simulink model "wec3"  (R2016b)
settings: Solver=ode4  StartTime=0  StopTime=500  FixedStep=0.01  MaxStep=0.01  RelTol=1e-3  EnableMultiTasking=on
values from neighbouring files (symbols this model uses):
  arAdaptiveLawData = 1/2*zModelSimple.zModelPto.arFreq.*     zModelSimple.zModelPto.arMagnitude./     cos(zModelSimple.zModelPto.arPhase*pi/180+pi/2)    [IMPACT_Control.m]
  arControllerRampGain = [0,0,1,1]    [IMPACT_Control.m]
  arControllerRampTime = [0 rStartRampTime rStartRampTime+rRampTimeLength 8000]    [IMPACT_Control.m]
  arEkfInitialisation = zeros(1,11)    [IMPACT_Control.m]
  arFrequency = zModelSimple.zModelPto.arFreq    [IMPACT_Control.m]
  arFrequencyRange = zModelSimple.zModelPto.arFreq    [IMPACT_Control.m]
  arImpedance = 1./zModelSimple.zModelPto.arMagnitude./zModelSimple.zModelPto.arFreq    [IMPACT_Control.m]
  arReferenceSpeedGain = [0.949075	0.948701	0.948086	0.947210	0.946078	0.944687	0.943012	0.941068	0.938816	0.936271	0.933396     0.930175	0.926598	0.922654	0.918263	0.913405	0.908086	0.901638	0.895829	0.888757	0.880863	0.872271	0.862778	0.852482     0.840874	0.827739	0.813322	0.797269	0.779501	0.760223	0.737472	0.712445	0.683207	0.651238	0.615591	0.577044	0.538330     0.488567	0.439533	0.392319	0.349558	0.318508	0.304192	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    [wec3AdditionalParams.m]
  iAdaptiveDamping = 0    [wec3_IMPACT_Project.m]    (also in IMPACT_Control.m = handles.iAdaptiveDamping; wec1_IMPACT_Project.m; wec2_IMPACT_Project.m; wec4IMPACT_Project.m)
  iControlType = 1    [wec3_IMPACT_Project.m]    (also in IMPACT_Control.m = handles.iControlType; wec1_IMPACT_Project.m; wec2_IMPACT_Project.m; wec4IMPACT_Project.m = 2)
  iPtoPositionConstraint = 1    [wec3_IMPACT_Project.m]    (also in IMPACT_Control.m = handles.iPtoPositionConstraint; wec1_IMPACT_Project.m = 0; wec2_IMPACT_Project.m; wec4IMPACT_Project.m)
  iSensorNoise = 0    [IMPACT_Control.m]
  m = m+1    (= 2)    [checkParamFile.m]
  rCogFloater = -0.7    [wec3_IMPACT_Model.m]    (also in wec3_IMPACT_Model2.m; paramInitial.m = get( handles.edit_rCogFloater, 'String' ); wec1_IMPACT_Model.m = -18; wec2_IMPACT_Model.m = -8.5)
  rCogSpar = -21.3    [wec3_IMPACT_Model.m]    (also in wec3_IMPACT_Model2.m; paramInitial.m = get( handles.edit_rCogSpar, 'String' ); wec4_IMPACT_Model.m = -36.6)
  rDisplacementLimit = 3.000000    (= 3)    [wec3_IMPACT_Project.m]    (also in IMPACT_Control.m = getValue(handles.edit_displacementLimit); wec1_IMPACT_Project.m = 10; wec2_IMPACT_Project.m = 10; wec4IMPACT_Project.m = 10)
  rGainForAntiWIndUp = tfControllerDiscrete.rGain    [IMPACT_Control.m]
  rMaxForcePto = 1000000000.000000    (= 1000000000)    [wec3_IMPACT_Project.m]    (also in IMPACT_Control.m = getValue(handles.edit_maxForcePto); wec1_IMPACT_Project.m = 1e+15; wec2_IMPACT_Project.m = 1e+15; wec4IMPACT_Project.m = 300000000)
  rMinForcePto = -1000000000.000000    (= -1000000000)    [wec3_IMPACT_Project.m]    (also in IMPACT_Control.m = getValue(handles.edit_minForcePto); wec1_IMPACT_Project.m = -1e+15; wec2_IMPACT_Project.m = -1e+15; wec4IMPACT_Project.m = -300000000)
  rOutputSampleTime = 0.010000    (= 0.01)    [wec3_IMPACT_Project.m]    (also in IMPACT_Control.m = getValue(handles.edit_outputSampleTime); wec1_IMPACT_Project.m; wec2_IMPACT_Project.m; wec4IMPACT_Project.m)
  rPassiveDampingGain = -519390.000000    (= -519390)    [wec3_IMPACT_Project.m]    (also in IMPACT_Control.m = getValue(handles.edit_gainPLD); wec1_IMPACT_Project.m = -214018.1537; wec2_IMPACT_Project.m = -1948070; wec4IMPACT_Project.m = -604830)
  s = tf('s')    [wec3_IMPACT_Model.m]    (also in wec3_IMPACT_Model2.m; IMPACT_Control.m; wec1_IMPACT_Model.m; wec2_IMPACT_Model.m)
  simu = simulationClass()    [wecSimInputFile.m]
  Z = magPhaseToComplex(zModelTf)    [IMPACT_Control.m]
undefined symbols (not defined in the file or in its folder): arControllerDiscreteDen, arControllerDiscreteNum, arExcForceFloaterDen, arExcForceFloaterNum, arExcForceSparDen, arExcForceSparNum, arFexcFloaterDen, arFexcFloaterNum, arFexcSparDen, arFexcSparNum, arRefeneceSpeedFreq, body, constraint, magnitude, mooring, N, pto, rAccelerationGainFloater, rAccelerationGainSpar, rBuoyancyGainFloater, rBuoyancyGainSpar, rDampingGainFloater, rDampingGainSpar, X, Y
libraries: nesl_utility x9, simulink x6, WECSim_Lib x5, sm_lib x5

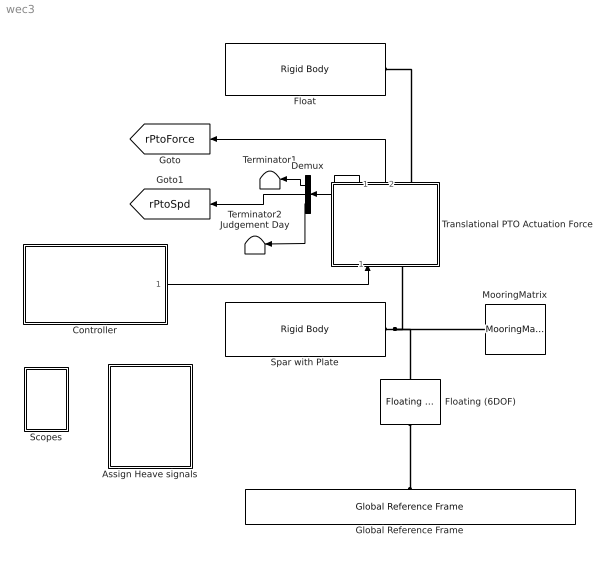
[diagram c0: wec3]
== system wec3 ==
  Assign Heave signals : Subsystem
  Controller : Subsystem
  Demux : Demux  Outputs=3
  Float : WECSim_Lib/Body Elements/Rigid Body  body=body(1)
  Floating (6DOF) : WECSim_Lib/Constraints/Floating (6DOF)  constraint=constraint(1)
  Global Reference Frame : WECSim_Lib/Frames/Global Reference Frame  waves=waves  simu=simu
  MooringMatrix : WECSim_Lib/Moorings/MooringMatrix  mooring=mooring(1)
  Scopes : Subsystem
  Spar with Plate : WECSim_Lib/Body Elements/Rigid Body  body=body(2)
  Terminator1 : Terminator
  Terminator2 Judgement Day : Terminator
  Translational PTO Actuation Force : Subsystem  AncestorBlock=WECSim_Lib/PTOs/Translational PTO Actuation Force
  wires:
  Translational PTO Actuation Force/2(ptoForce) -> [rPtoForce]
  Controller/1(forceDemandOut) -> Translational PTO Actuation Force/1(Force)
  Translational PTO Actuation Force/1(Response) -> Demux/1
  Demux/2 -> [rPtoSpd]
  Demux/1 -> Terminator1/1
  Demux/3 -> Terminator2 Judgement Day/1
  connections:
  Spar with Plate/RConn1 -- Translational PTO Actuation Force/LConn1 -- Floating (6DOF)/RConn1 -- MooringMatrix/LConn1
  Translational PTO Actuation Force/RConn1 -- Float/RConn1
  Floating (6DOF)/LConn1 -- Global Reference Frame/RConn1

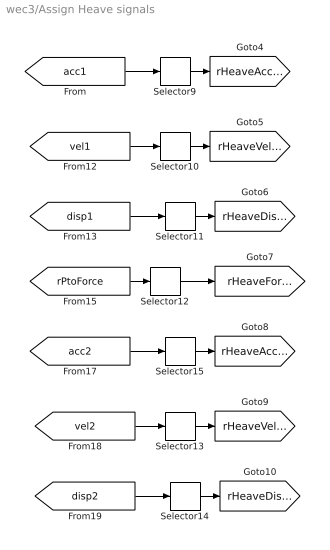
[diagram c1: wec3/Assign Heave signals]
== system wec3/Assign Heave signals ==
  Selector{9..15} (7 alike) : Selector  InputPortWidth=6  IndexOptions=Index vector (dialog)  Indices=3  OutputSizes=1
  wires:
  Selector11/1 -> [rHeaveDispFl]
  [disp1] -> Selector11/1
  Selector12/1 -> [rHeaveForcePto]
  [vel1] -> Selector10/1
  [acc1] -> Selector9/1
  Selector10/1 -> [rHeaveVelFl]
  Selector9/1 -> [rHeaveAccFl]
  [rPtoForce] -> Selector12/1
  Selector14/1 -> [rHeaveDispSp]
  Selector13/1 -> [rHeaveVelSp]
  [vel2] -> Selector13/1
  [disp2] -> Selector14/1
  [acc2] -> Selector15/1
  Selector15/1 -> [rHeaveAccSp]

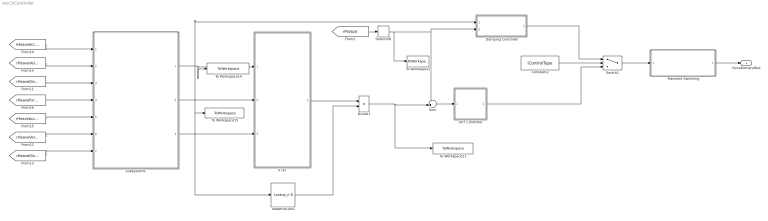
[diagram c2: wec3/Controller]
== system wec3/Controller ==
  Constant2 : Constant  Value=iControlType
  Damping Controller : Subsystem
  Divide1 : Product  Inputs=**
  OVT Controller : Subsystem
  Selector6 : Selector  InputPortWidth=6  IndexOptions=Index vector (dialog)  Indices=3  OutputSizes=1
  Subsystem1 : Subsystem
  Sum : Sum  Inputs=-+|
  Switch1 : Switch  Threshold=2
  To Workspace14 : ToWorkspace  VariableName=arCombinedExcForce  SampleTime=simu.dtOut
  To Workspace15 : ToWorkspace  VariableName=arFreqCombExcF  SampleTime=simu.dtOut
  To Workspace2 : ToWorkspace  VariableName=arPtoVelocity  SampleTime=0.05
  To Workspace21 : ToWorkspace  VariableName=arReferenceVelocity  SampleTime=simu.dtOut
  Transient Switching : Subsystem
  "V ref " : Subsystem
  adaptiveLaw1 : Lookup_n-D  NumberOfTableDimensions=1  BreakpointsForDimension1=arRefeneceSpeedFreq  Table=arReferenceSpeedGain  InternalRulePriority=Speed  RndMeth=Simplest
  forceDemandOut : Outport
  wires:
  [rHeaveDispSp] -> Subsystem1/7(sparPos)
  [rHeaveVelFl] -> Subsystem1/2(floaterVel)
  [rHeaveAccFl] -> Subsystem1/1(floaterAcc)
  [rHeaveAccSp] -> Subsystem1/5(sparAcc)
  [rHeaveVelSp] -> Subsystem1/6(sparVel)
  [rHeaveForcePto] -> Subsystem1/4(ptoForce)
  [rHeaveDispFl] -> Subsystem1/3(floaterPos)
  Damping Controller/1(forceDemand) -> Switch1/1
  Switch1/1 -> Transient Switching/1(forceDemandIn)
  Constant2/1 -> Switch1/2
  OVT Controller/1(forceDemand) -> Switch1/3
  Sum/1 -> OVT Controller/1(error)
  Selector6/1 -> To Workspace2/1, Sum/1, Damping Controller/2(velocity)
  [rPtoSpd] -> Selector6/1
  Subsystem1/2(Frequency) -> adaptiveLaw1/1, To Workspace15/1, "V ref "/2(ekfFrequency), Damping Controller/1(ekfFrequency)
  Subsystem1/3(Exc. Force Amplitude) -> "V ref "/3(ekfAmplitude)
  Subsystem1/1(Combined Excitation Force) -> To Workspace14/1, "V ref "/1(phiOut)
  Transient Switching/1(forceDemandOut) -> forceDemandOut/1
  "V ref "/1(referenceVelocity) -> Divide1/1
  adaptiveLaw1/1 -> Divide1/2
  Divide1/1 -> To Workspace21/1, Sum/2

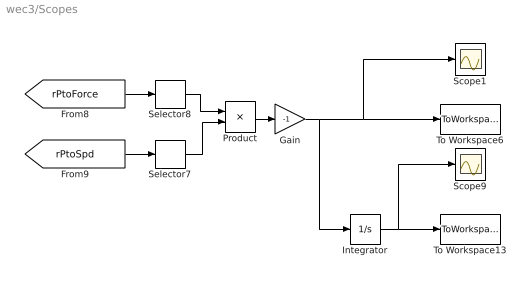
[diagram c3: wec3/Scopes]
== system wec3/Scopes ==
  Gain : Gain  Gain=-1
  Integrator : Integrator
  Product : Product
  Scope1 : Scope
  Scope9 : Scope
  Selector7 : Selector  InputPortWidth=6  IndexOptions=Index vector (dialog)  Indices=3  OutputSizes=1
  Selector8 : Selector  InputPortWidth=6  IndexOptions=Index vector (dialog)  Indices=3  OutputSizes=1
  To Workspace13 : ToWorkspace  VariableName=arWecEnergy  SampleTime=simu.dtOut
  To Workspace6 : ToWorkspace  VariableName=arWecPower  SampleTime=simu.dtOut
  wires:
  Gain/1 -> To Workspace6/1, Scope1/1, Integrator/1
  [rPtoForce] -> Selector8/1
  [rPtoSpd] -> Selector7/1
  Product/1 -> Gain/1
  Selector7/1 -> Product/2
  Selector8/1 -> Product/1
  Integrator/1 -> Scope9/1, To Workspace13/1

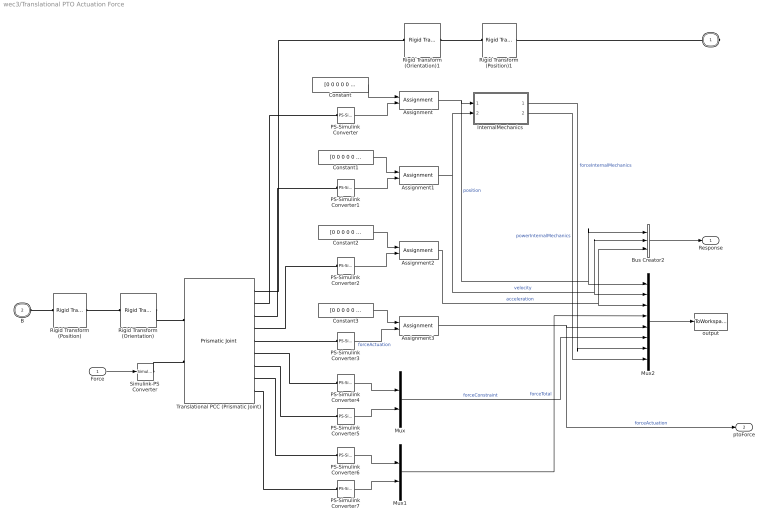
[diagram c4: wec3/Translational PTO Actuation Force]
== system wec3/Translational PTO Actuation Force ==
  Force : Inport
  Assignment{,1..3} (4 alike) : Assignment  IndexOptions=Index vector (dialog)  Indices=3  OutputSizes=1
  Bus Creator2 : BusCreator  Inputs=3
  Constant{,1..3} (4 alike) : Constant  Value=[0 0 0 0 0 0]
  InternalMechanics : Subsystem
  Mux : Mux  Inputs=2
  Mux1 : Mux  Inputs=2
  Mux2 : Mux  Inputs=8
  PS-Simulink Converter{,1..7} (8 alike) : nesl_utility/PS-Simulink Converter  PhysicalDomain=network_engine_domain  SubClassName=ps_output  LeftPortType=input  RightPortType=output  PseudoPeriodic=off  Frequencies=[]  Unit=1  AffineConversion=off
  Rigid Transform (Position) : sm_lib/Frames and Transforms/Rigid Transform  TranslationMethod=Cartesian  TranslationStandardOffset=0  TranslationLengthUnit=m  TranslationStandardAxis=+Z  TranslationCartesianOffset=pto.initDisp.initLinDisp + pto.loc  TranslationROffset=0  TranslationROffsetUnits=m  TranslationZOffset=0  TranslationZOffsetUnits=m  TranslationThetaOffset=0  TranslationThetaOffsetUnits=deg  RotationMethod=None  RotationAngleUnits=rad  RotationStandardAxis=+Y  RotationAngle=0  RotationArbitraryAxis=[0 1 0]  FollAlignAxisA=+X  BaseAlignAxisA=+Y  FollAlignAxisB=+Y  BaseAlignAxisB=+Z  RotationSequenceAxes=FollowerAxes  RotationSequence=XYX  RotationSequenceAngles=[0 0 0]  RotationSequenceAnglesUnits=deg  RotationMatrix=[1 0 0; 0 1 0; 0 0 1]
  Rigid Transform (Position)1 : sm_lib/Frames and Transforms/Rigid Transform  TranslationMethod=Cartesian  TranslationStandardOffset=0  TranslationLengthUnit=m  TranslationStandardAxis=+Z  TranslationCartesianOffset=pto.initDisp.initLinDisp + pto.loc  TranslationROffset=0  TranslationROffsetUnits=m  TranslationZOffset=0  TranslationZOffsetUnits=m  TranslationThetaOffset=0  TranslationThetaOffsetUnits=deg  RotationMethod=None  RotationAngleUnits=rad  RotationStandardAxis=+Y  RotationAngle=0  RotationArbitraryAxis=[0 1 0]  FollAlignAxisA=+X  BaseAlignAxisA=+Y  FollAlignAxisB=+Y  BaseAlignAxisB=+Z  RotationSequenceAxes=FollowerAxes  RotationSequence=XYX  RotationSequenceAngles=[0 0 0]  RotationSequenceAnglesUnits=deg  RotationMatrix=[1 0 0; 0 1 0; 0 0 1]
  Rigid Transform (Orientation) : sm_lib/Frames and Transforms/Rigid Transform  TranslationMethod=None  TranslationStandardOffset=0  TranslationLengthUnit=m  TranslationStandardAxis=+Z  TranslationCartesianOffset=0  TranslationROffset=0  TranslationROffsetUnits=m  TranslationZOffset=0  TranslationZOffsetUnits=m  TranslationThetaOffset=0  TranslationThetaOffsetUnits=deg  RotationMethod=RotationMatrix  RotationAngleUnits=rad  RotationStandardAxis=+Y  RotationAngle=0  RotationArbitraryAxis=[0 1 0]  FollAlignAxisA=+X  BaseAlignAxisA=+Y  FollAlignAxisB=+Y  BaseAlignAxisB=+Z  RotationSequenceAxes=FollowerAxes  RotationSequence=XYX  RotationSequenceAngles=[0 0 0]  RotationSequenceAnglesUnits=deg  RotationMatrix=pto.orientation.rotationMatrix
  Rigid Transform (Orientation)1 : sm_lib/Frames and Transforms/Rigid Transform  TranslationMethod=None  TranslationStandardOffset=0  TranslationLengthUnit=m  TranslationStandardAxis=+Z  TranslationCartesianOffset=0  TranslationROffset=0  TranslationROffsetUnits=m  TranslationZOffset=0  TranslationZOffsetUnits=m  TranslationThetaOffset=0  TranslationThetaOffsetUnits=deg  RotationMethod=RotationMatrix  RotationAngleUnits=rad  RotationStandardAxis=+Y  RotationAngle=0  RotationArbitraryAxis=[0 1 0]  FollAlignAxisA=+X  BaseAlignAxisA=+Y  FollAlignAxisB=+Y  BaseAlignAxisB=+Z  RotationSequenceAxes=FollowerAxes  RotationSequence=XYX  RotationSequenceAngles=[0 0 0]  RotationSequenceAnglesUnits=deg  RotationMatrix=pto.orientation.rotationMatrix
  Simulink-PS Converter : nesl_utility/Simulink-PS Converter  PhysicalDomain=network_engine_domain  SubClassName=ps_input  LeftPortType=input  RightPortType=output  PseudoPeriodic=off  Frequencies=[]  NoiseDistribution=none  NoiseParameters=[]  Unit=1  AffineConversion=off  InputFiltering=off  SimscapeFilterOrder=1  InputFilterTimeConstant=0.001  UdotUserProvided=1
  Translational PCC (Prismatic Joint) : sm_lib/Joints/Prismatic Joint  SenseConstraintForce=on  SenseConstraintForceX=off  SenseConstraintForceY=off  SenseConstraintForceZ=off  SenseConstraintTorque=on  SenseConstraintTorqueX=off  SenseConstraintTorqueY=off  SenseConstraintTorqueZ=off  SenseTotalForce=on  SenseTotalForceX=off  SenseTotalForceY=off  SenseTotalForceZ=off  SenseTotalTorque=on  SenseTotalTorqueX=off  SenseTotalTorqueY=off  SenseTotalTorqueZ=off  CompositeWrenchDir=BaseOnFollower  CompositeWrenchFrame=BaseFrame  EquilibriumPosition=0  EquilibriumPositionUnits=m  SpringStiffness=pto.k  SpringStiffnessUnits=N/m  DampingCoefficient=pto.c  DampingCoefficientUnits=N/(m/s)  TorqueActuationMode=InputTorque  MotionActuationMode=ComputedMotion  SensePosition=on  SenseVelocity=on  SenseAcceleration=on  SenseTorqueForce=on  PositionTargetSpecify=off  PositionTargetPriority=High  PositionTargetValue=0  PositionTargetValueUnits=m  VelocityTargetSpecify=off  VelocityTargetPriority=High  VelocityTargetValue=0  VelocityTargetValueUnits=m/s
  output : ToWorkspace  VariableName=pto1_out  SaveFormat=Structure With Time  SampleTime=-1
  F : PMIOPort  Port=1  Side=Right
  B : PMIOPort  Port=2  Side=Left
  Response : Outport
  ptoForce : Outport  Port=2
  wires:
  Bus Creator2/1 -> Response/1
  Assignment/1 -> Mux2/1, Bus Creator2/1, InternalMechanics/1(Position)  "position"
  Assignment1/1 -> Mux2/2, Bus Creator2/2, InternalMechanics/2(Velocity)  "velocity"
  Assignment2/1 -> Mux2/3, Bus Creator2/3  "acceleration"
  Force/1 -> Simulink-PS Converter/1
  Mux2/1 -> output/1
  Mux/1 -> Mux2/6  "forceConstraint"
  Mux1/1 -> Mux2/4  "forceTotal"
  PS-Simulink Converter4/1 -> Mux/1
  PS-Simulink Converter5/1 -> Mux/2
  PS-Simulink Converter6/1 -> Mux1/1
  PS-Simulink Converter7/1 -> Mux1/2
  Assignment3/1 -> ptoForce/1, Mux2/5  "forceActuation"
  Constant/1 -> Assignment/1
  PS-Simulink Converter/1 -> Assignment/2
  Constant1/1 -> Assignment1/1
  PS-Simulink Converter1/1 -> Assignment1/2
  Constant2/1 -> Assignment2/1
  PS-Simulink Converter2/1 -> Assignment2/2
  InternalMechanics/1(Force) -> Mux2/7  "forceInternalMechanics"
  InternalMechanics/2(Power) -> Mux2/8  "powerInternalMechanics"
  Constant3/1 -> Assignment3/1
  PS-Simulink Converter3/1 -> Assignment3/2  "forceActuation"
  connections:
  Rigid Transform (Position)/RConn1 -- Rigid Transform (Orientation)/LConn1
  Rigid Transform (Position)1/RConn1 -- Rigid Transform (Orientation)1/LConn1
  Simulink-PS Converter/RConn1 -- Translational PCC (Prismatic Joint)/LConn2
  Rigid Transform (Orientation)/RConn1 -- Translational PCC (Prismatic Joint)/LConn1
  Rigid Transform (Position)/LConn1 -- B/RConn1
  Translational PCC (Prismatic Joint)/RConn5 -- PS-Simulink Converter3/LConn1
  Translational PCC (Prismatic Joint)/RConn9 -- PS-Simulink Converter7/LConn1
  Rigid Transform (Orientation)1/RConn1 -- Translational PCC (Prismatic Joint)/RConn1
  Translational PCC (Prismatic Joint)/RConn4 -- PS-Simulink Converter2/LConn1
  Translational PCC (Prismatic Joint)/RConn7 -- PS-Simulink Converter5/LConn1
  Translational PCC (Prismatic Joint)/RConn3 -- PS-Simulink Converter1/LConn1
  Rigid Transform (Position)1/LConn1 -- F/RConn1
  Translational PCC (Prismatic Joint)/RConn8 -- PS-Simulink Converter6/LConn1
  Translational PCC (Prismatic Joint)/RConn2 -- PS-Simulink Converter/LConn1
  Translational PCC (Prismatic Joint)/RConn6 -- PS-Simulink Converter4/LConn1

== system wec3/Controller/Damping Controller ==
  ekfFrequency : Inport
  velocity : Inport  Port=2
  Constant2 : Constant  Value=iAdaptiveDamping
  Divide2 : Product  Inputs=**
  Gain6 : Gain  Gain=rPassiveDampingGain
  Gain7 : Gain  Gain=-1
  Switch1 : Switch  Criteria=u2 > Threshold
  adaptiveLaw1 : Lookup_n-D  NumberOfTableDimensions=1  BreakpointsForDimension1=arFrequency  Table=arImpedance  InternalRulePriority=Speed  RndMeth=Simplest
  forceDemand : Outport
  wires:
  Divide2/1 -> Switch1/1
  ekfFrequency/1 -> adaptiveLaw1/1
  adaptiveLaw1/1 -> Gain7/1
  Constant2/1 -> Switch1/2
  Switch1/1 -> forceDemand/1
  Gain7/1 -> Divide2/1
  velocity/1 -> Divide2/2, Gain6/1
  Gain6/1 -> Switch1/3

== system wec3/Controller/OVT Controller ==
  error : Inport
  Anti wind-up controller : Subsystem
  forceDemand : Outport
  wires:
  error/1 -> Anti wind-up controller/1(error)
  Anti wind-up controller/1(Out1) -> forceDemand/1

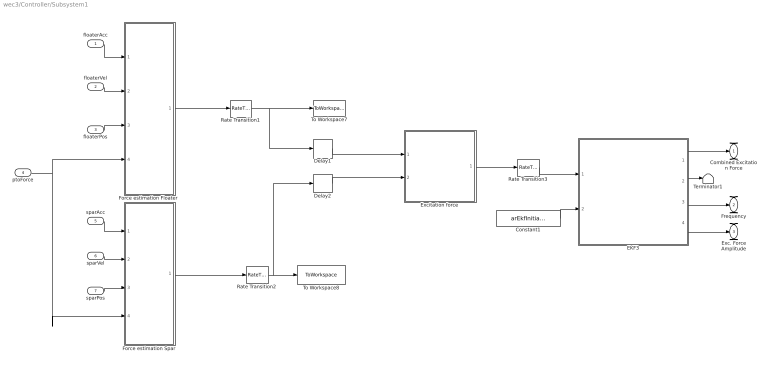
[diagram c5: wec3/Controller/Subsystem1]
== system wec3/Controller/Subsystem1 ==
  floaterAcc : Inport
  floaterVel : Inport  Port=2
  floaterPos : Inport  Port=3
  ptoForce : Inport  Port=4
  sparAcc : Inport  Port=5
  sparVel : Inport  Port=6
  sparPos : Inport  Port=7
  Constant1 : Constant  Value=arEkfInitialisation
  Delay1 : Delay  DelayLength=1  SampleTime=simu.dt
  Delay2 : Delay  DelayLength=1  SampleTime=simu.dt
  EKF3 : MATLAB Function  TreatAsAtomicUnit=on
  Excitation force : Subsystem
  "Force estimation Floater " : Subsystem
  Force estimation Spar : Subsystem
  Rate Transition1 : RateTransition  OutPortSampleTimeMultiple=0.01  OutPortSampleTime=rKalmanFilterSampleTime
  Rate Transition2 : RateTransition  OutPortSampleTimeMultiple=0.01  OutPortSampleTime=rKalmanFilterSampleTime
  Rate Transition3 : RateTransition  OutPortSampleTimeMultiple=0.01  OutPortSampleTime=rKalmanFilterSampleTime
  Terminator1 : Terminator
  To Workspace7 : ToWorkspace  VariableName=arExcForceFl  SampleTime=simu.dtOut
  To Workspace8 : ToWorkspace  VariableName=arExcForceSp  SampleTime=simu.dtOut
  Combined Excitation Force : Outport
  Frequency : Outport  Port=2
  Exc. Force Amplitude : Outport  Port=3
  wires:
  Excitation force/1(Combined Fexc) -> Rate Transition3/1
  Rate Transition2/1 -> Delay2/1, To Workspace8/1
  ptoForce/1 -> Force estimation Spar/4(PTO Force), "Force estimation Floater "/4(PTO force)
  floaterVel/1 -> "Force estimation Floater "/2(Velocity)
  sparVel/1 -> Force estimation Spar/2(Velocity)
  Rate Transition1/1 -> To Workspace7/1, Delay1/1
  sparAcc/1 -> Force estimation Spar/1(Acceleration)
  sparPos/1 -> Force estimation Spar/3(Position)
  floaterAcc/1 -> "Force estimation Floater "/1(Acceleration)
  floaterPos/1 -> "Force estimation Floater "/3(Position)
  "Force estimation Floater "/1(excForce) -> Rate Transition1/1
  Force estimation Spar/1(excForce) -> Rate Transition2/1
  Rate Transition3/1 -> EKF3/1(rEstimatedExcitationForce)
  EKF3/3(rFrequencyOutput) -> Frequency/1
  EKF3/4(rAmplitudeOutput) -> Exc. Force Amplitude/1
  EKF3/1(rPhi0Output) -> Combined Excitation Force/1
  Constant1/1 -> EKF3/2(arEkfInitialisation)
  EKF3/2(rPhi0StarOutput) -> Terminator1/1
  Delay1/1 -> Excitation force/1(Fexc floater)
  Delay2/1 -> Excitation force/2(Fexc spar)

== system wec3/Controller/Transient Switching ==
  forceDemandIn : Inport
  Constant : Constant
  IC : InitialCondition  Value=0
  Product : Product
  To Workspace3 : ToWorkspace  VariableName=arForceDemand  SampleTime=rOutputSampleTime
  To Workspace7 : ToWorkspace  VariableName=arForceDemandIn  SampleTime=rOutputSampleTime
  forceDemandOut : Outport
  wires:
  forceDemandIn/1 -> Product/2, To Workspace7/1
  Product/1 -> IC/1
  IC/1 -> To Workspace3/1, forceDemandOut/1
  Constant/1 -> Product/1

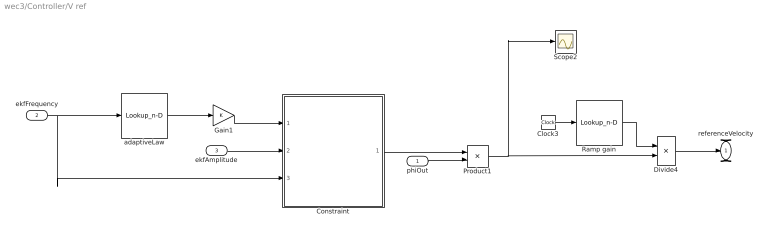
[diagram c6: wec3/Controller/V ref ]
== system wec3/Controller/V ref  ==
  phiOut : Inport
  ekfFrequency : Inport  Port=2
  ekfAmplitude : Inport  Port=3
  Clock3 : Clock
  Constraint : Subsystem
  Divide4 : Product  Inputs=**
  Gain1 : Gain
  Product1 : Product
  Ramp gain : Lookup_n-D  NumberOfTableDimensions=1  BreakpointsForDimension1=arControllerRampTime  Table=arControllerRampGain  InternalRulePriority=Speed  RndMeth=Simplest
  Scope2 : Scope
  adaptiveLaw : Lookup_n-D  NumberOfTableDimensions=1  BreakpointsForDimension1=arFrequencyRange  Table=arAdaptiveLawData  InternalRulePriority=Speed  RndMeth=Simplest
  referenceVelocity : Outport
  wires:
  Constraint/1(referenceVelocity) -> Product1/1
  Ramp gain/1 -> Divide4/1
  Clock3/1 -> Ramp gain/1
  Gain1/1 -> Constraint/1(1/2B)
  adaptiveLaw/1 -> Gain1/1
  Divide4/1 -> referenceVelocity/1
  ekfFrequency/1 -> Constraint/3(ekfFrequency), adaptiveLaw/1
  ekfAmplitude/1 -> Constraint/2(Amp)
  Product1/1 -> Scope2/1, Divide4/2
  phiOut/1 -> Product1/2

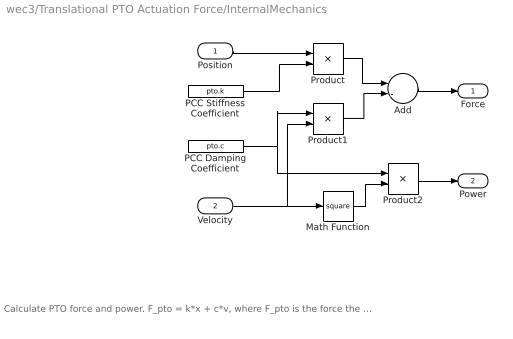
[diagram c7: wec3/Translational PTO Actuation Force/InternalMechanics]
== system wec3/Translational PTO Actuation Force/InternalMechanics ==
  note: Calculate PTO force and power. F_pto = k*x + c*v, where F_pto is the force the PTO applies to the body (at the PTO location), x and v are the joint position and velocity. The power extracted is P = c * v^2
  Position : Inport
  Velocity : Inport  Port=2
  Add : Sum  Inputs=--
  Math Function : Math  Operator=square
  PCC Damping Coefficient : Constant  Value=pto.c
  PCC Stiffness Coefficient : Constant  Value=pto.k
  Product : Product  Inputs=**
  Product1 : Product  Inputs=**
  Product2 : Product  Inputs=**
  Force : Outport
  Power : Outport  Port=2
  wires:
  PCC Damping Coefficient/1 -> Product2/1, Product1/1
  Product2/1 -> Power/1
  Velocity/1 -> Math Function/1, Product1/2
  PCC Stiffness Coefficient/1 -> Product/2
  Position/1 -> Product/1
  Add/1 -> Force/1
  Math Function/1 -> Product2/2
  Product/1 -> Add/1
  Product1/1 -> Add/2

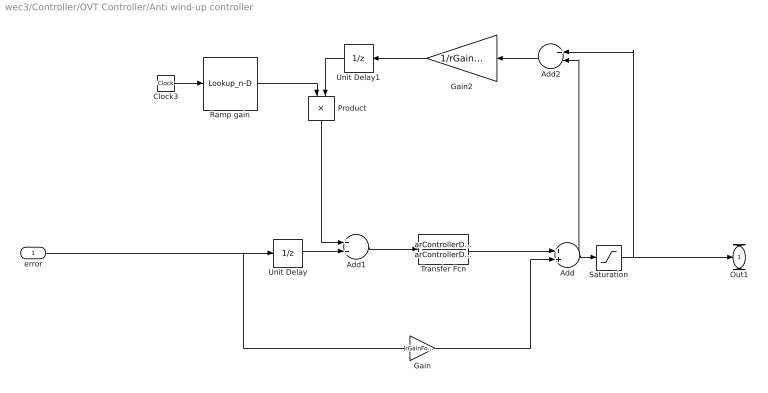
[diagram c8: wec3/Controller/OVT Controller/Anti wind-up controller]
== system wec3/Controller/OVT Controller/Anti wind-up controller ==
  error : Inport
  Add : Sum
  Add1 : Sum
  Add2 : Sum  Inputs=+-
  Clock3 : Clock
  Gain : Gain  Gain=rGainForAntiWIndUp
  Gain2 : Gain  Gain=1/rGainForAntiWIndUp
  Product : Product
  Ramp gain : Lookup_n-D  NumberOfTableDimensions=1  BreakpointsForDimension1=arControllerRampTime  Table=arControllerRampGain  InternalRulePriority=Speed  RndMeth=Simplest
  Saturation : Saturate  UpperLimit=rMaxForcePto  LowerLimit=rMinForcePto
  Transfer Fcn : TransferFcn  Numerator=arControllerDiscreteNum  Denominator=arControllerDiscreteDen
  Unit Delay : UnitDelay  SampleTime=0.01
  Unit Delay1 : UnitDelay  SampleTime=0.01
  Out1 : Outport
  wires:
  Add/1 -> Saturation/1, Add2/2
  Gain/1 -> Add/2
  Unit Delay/1 -> Add1/2
  Gain2/1 -> Unit Delay1/1
  error/1 -> Gain/1, Unit Delay/1
  Add2/1 -> Gain2/1
  Add1/1 -> Transfer Fcn/1
  Clock3/1 -> Ramp gain/1
  Ramp gain/1 -> Product/1
  Product/1 -> Add1/1
  Unit Delay1/1 -> Product/2
  Saturation/1 -> Out1/1, Add2/1
  Transfer Fcn/1 -> Add/1

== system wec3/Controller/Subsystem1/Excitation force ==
  Fexc floater : Inport
  Fexc spar : Inport  Port=2
  Add : Sum
  Scope : Scope
  Scope1 : Scope
  Scope2 : Scope
  Transfer Fcn : TransferFcn  Numerator=arFexcFloaterNum  Denominator=arFexcFloaterDen
  Transfer Fcn1 : TransferFcn  Numerator=arFexcSparNum  Denominator=arFexcSparDen
  Combined Fexc : Outport
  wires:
  Fexc floater/1 -> Transfer Fcn/1
  Fexc spar/1 -> Transfer Fcn1/1
  Transfer Fcn/1 -> Add/1, Scope1/1
  Transfer Fcn1/1 -> Add/2, Scope2/1
  Add/1 -> Combined Fexc/1, Scope/1

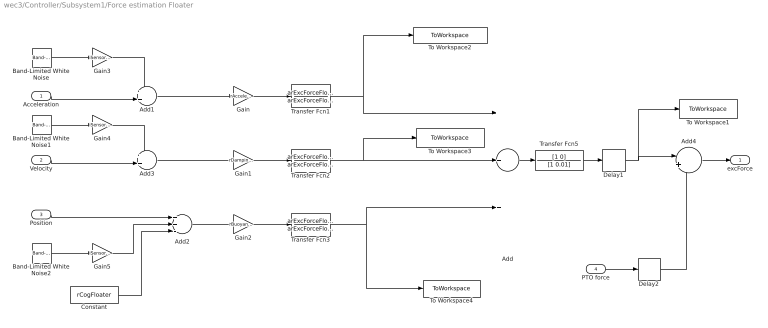
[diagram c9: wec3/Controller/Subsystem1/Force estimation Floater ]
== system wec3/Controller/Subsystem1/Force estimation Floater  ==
  Acceleration : Inport
  Velocity : Inport  Port=2
  Position : Inport  Port=3
  PTO force : Inport  Port=4
  Add : Sum  Inputs=+++
  Add1 : Sum  Inputs=++|
  Add2 : Sum  Inputs=++-
  Add3 : Sum  Inputs=++|
  Add4 : Sum  Inputs=|+-
  Band-Limited White Noise : simulink/Sources/Band-Limited White Noise  Cov=[0.1]  Ts=simu.dt  seed=[23341]
  Band-Limited White Noise1 : simulink/Sources/Band-Limited White Noise  Cov=[0.1]  Ts=simu.dt  seed=[23341]
  Band-Limited White Noise2 : simulink/Sources/Band-Limited White Noise  Cov=[0.1]  Ts=simu.dt  seed=[23341]
  Constant : Constant  Value=rCogFloater
  Delay1 : Delay  DelayLength=1  SampleTime=simu.dt
  Delay2 : Delay  DelayLength=1  SampleTime=simu.dt
  Gain : Gain  Gain=rAccelerationGainFloater
  Gain1 : Gain  Gain=rDampingGainFloater
  Gain2 : Gain  Gain=rBuoyancyGainFloater
  Gain3 : Gain  Gain=iSensorNoise
  Gain4 : Gain  Gain=iSensorNoise
  Gain5 : Gain  Gain=iSensorNoise
  To Workspace1 : ToWorkspace  VariableName=arInertialForceFl  SampleTime=rOutputSampleTime
  To Workspace2 : ToWorkspace  VariableName=arAccComponentFl  SampleTime=rOutputSampleTime
  To Workspace3 : ToWorkspace  VariableName=arVelComponentFl  SampleTime=rOutputSampleTime
  To Workspace4 : ToWorkspace  VariableName=arPosComponentFl  SampleTime=rOutputSampleTime
  Transfer Fcn1 : TransferFcn  Numerator=arExcForceFloaterNum  Denominator=arExcForceFloaterDen
  Transfer Fcn2 : TransferFcn  Numerator=arExcForceFloaterNum  Denominator=arExcForceFloaterDen
  Transfer Fcn3 : TransferFcn  Numerator=arExcForceFloaterNum  Denominator=arExcForceFloaterDen
  Transfer Fcn5 : TransferFcn  Numerator=[1 0]  Denominator=[1 0.01]
  excForce : Outport
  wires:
  Acceleration/1 -> Add1/2
  Band-Limited White Noise/1 -> Gain3/1
  Gain5/1 -> Add2/2
  Add2/1 -> Gain2/1
  Gain2/1 -> Transfer Fcn3/1
  Gain1/1 -> Transfer Fcn2/1
  Gain/1 -> Transfer Fcn1/1
  Constant/1 -> Add2/3
  Gain4/1 -> Add3/1
  Add3/1 -> Gain1/1
  Gain3/1 -> Add1/1
  Velocity/1 -> Add3/2
  Add1/1 -> Gain/1
  Position/1 -> Add2/1
  Band-Limited White Noise1/1 -> Gain4/1
  Band-Limited White Noise2/1 -> Gain5/1
  Add4/1 -> excForce/1
  PTO force/1 -> Delay2/1
  Delay2/1 -> Add4/2
  Delay1/1 -> To Workspace1/1, Add4/1
  Transfer Fcn1/1 -> To Workspace2/1, Add/1
  Transfer Fcn2/1 -> To Workspace3/1, Add/2
  Transfer Fcn3/1 -> To Workspace4/1, Add/3
  Transfer Fcn5/1 -> Delay1/1
  Add/1 -> Transfer Fcn5/1

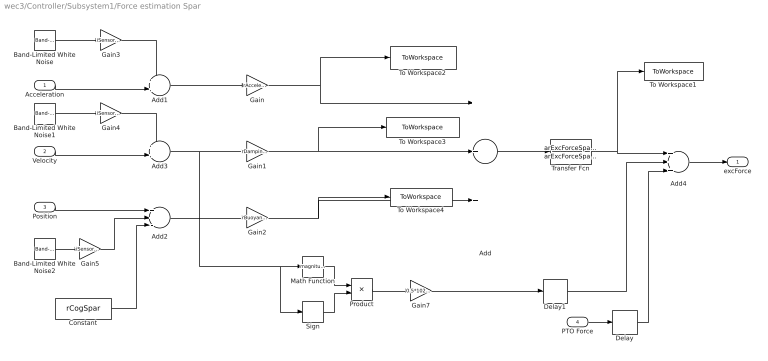
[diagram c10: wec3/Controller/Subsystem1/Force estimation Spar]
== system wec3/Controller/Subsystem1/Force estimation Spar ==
  Acceleration : Inport
  Velocity : Inport  Port=2
  Position : Inport  Port=3
  PTO Force : Inport  Port=4
  Add : Sum  Inputs=+++
  Add1 : Sum  Inputs=++|
  Add2 : Sum  Inputs=++-
  Add3 : Sum  Inputs=++|
  Add4 : Sum  Inputs=+++
  Band-Limited White Noise : simulink/Sources/Band-Limited White Noise  Cov=[0.1]  Ts=simu.dt  seed=[23341]
  Band-Limited White Noise1 : simulink/Sources/Band-Limited White Noise  Cov=[0.1]  Ts=simu.dt  seed=[23341]
  Band-Limited White Noise2 : simulink/Sources/Band-Limited White Noise  Cov=[0.1]  Ts=simu.dt  seed=[23341]
  Constant : Constant  Value=rCogSpar
  Delay : Delay  DelayLength=1  SampleTime=simu.dt
  Delay1 : Delay  DelayLength=1  SampleTime=simu.dt
  Gain : Gain  Gain=rAccelerationGainSpar
  Gain1 : Gain  Gain=rDampingGainSpar
  Gain2 : Gain  Gain=rBuoyancyGainSpar
  Gain3 : Gain  Gain=iSensorNoise
  Gain4 : Gain  Gain=iSensorNoise
  Gain5 : Gain  Gain=iSensorNoise
  Gain7 : Gain  Gain=0.5*1025*pi*15^2*4
  Math Function : Math  Operator=magnitude^2
  Product : Product
  Sign : Signum
  To Workspace1 : ToWorkspace  VariableName=arInertialForceSp  SampleTime=rOutputSampleTime
  To Workspace2 : ToWorkspace  VariableName=arAccComponentSp  SampleTime=rOutputSampleTime
  To Workspace3 : ToWorkspace  VariableName=arVelComponentSp  SampleTime=rOutputSampleTime
  To Workspace4 : ToWorkspace  VariableName=arPosComponentSp  SampleTime=rOutputSampleTime
  Transfer Fcn : TransferFcn  Numerator=arExcForceSparNum  Denominator=arExcForceSparDen
  excForce : Outport
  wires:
  Transfer Fcn/1 -> To Workspace1/1, Add4/1
  Add4/1 -> excForce/1
  Add/1 -> Transfer Fcn/1
  Delay/1 -> Add4/3
  Band-Limited White Noise2/1 -> Gain5/1
  Band-Limited White Noise1/1 -> Gain4/1
  Position/1 -> Add2/1
  Add1/1 -> Gain/1
  Velocity/1 -> Add3/2
  Gain3/1 -> Add1/1
  Add3/1 -> Sign/1, Math Function/1, Gain1/1
  Gain4/1 -> Add3/1
  Constant/1 -> Add2/3
  Gain/1 -> To Workspace2/1, Add/1
  Gain1/1 -> To Workspace3/1, Add/2
  Gain2/1 -> To Workspace4/1, Add/3
  PTO Force/1 -> Delay/1
  Add2/1 -> Gain2/1
  Gain5/1 -> Add2/2
  Band-Limited White Noise/1 -> Gain3/1
  Acceleration/1 -> Add1/2
  Math Function/1 -> Product/1
  Sign/1 -> Product/2
  Product/1 -> Gain7/1
  Gain7/1 -> Delay1/1
  Delay1/1 -> Add4/2

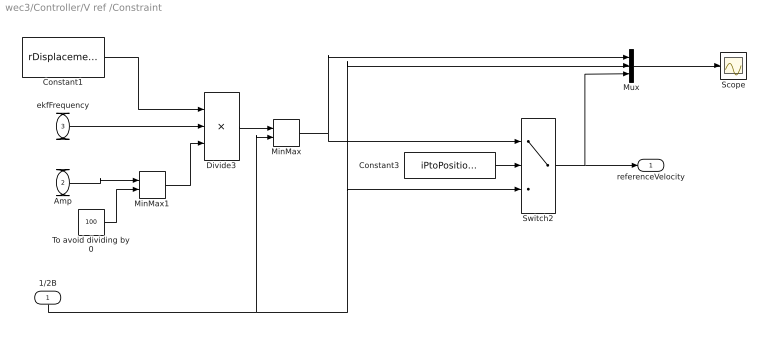
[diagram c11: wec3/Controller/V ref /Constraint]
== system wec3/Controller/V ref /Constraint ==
  1/2B : Inport
  Amp : Inport  Port=2
  ekfFrequency : Inport  Port=3
  Constant1 : Constant  Value=rDisplacementLimit
  Constant3 : Constant  Value=iPtoPositionConstraint
  Divide3 : Product  Inputs=**/
  MinMax : MinMax  Inputs=2
  MinMax1 : MinMax  Function=max  Inputs=2
  Mux : Mux  Inputs=3
  Scope : Scope
  Switch2 : Switch  Criteria=u2 > Threshold
  To avoid dividing by 0 : Constant  Value=100
  referenceVelocity : Outport
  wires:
  MinMax/1 -> Mux/1, Switch2/1
  ekfFrequency/1 -> Divide3/2
  Constant1/1 -> Divide3/1
  MinMax1/1 -> Divide3/3
  Divide3/1 -> MinMax/1
  To avoid dividing by 0/1 -> MinMax1/2
  Amp/1 -> MinMax1/1
  Constant3/1 -> Switch2/2
  Switch2/1 -> Mux/3, referenceVelocity/1
  Mux/1 -> Scope/1
  1/2B/1 -> MinMax/2, Switch2/3, Mux/2

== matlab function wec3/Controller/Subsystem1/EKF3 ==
function [rPhi0Output,rPhi0StarOutput,rFrequencyOutput, rAmplitudeOutput] = kalmanFilter(rEstimatedExcitationForce,arEkfInitialisation)

%%%%%%%%%%%%%%%%%%%%%%%%%%%%%%%%%%%%%%%%%%%%%%%%%%%%%%%%%%%%%%%%%%%%%%%%%
%%%                     Extended Kalman Filter                        %%%

%-----------------------------
% State equations
% X[n+1] = A*X[n] + B*U[n] + v
% Output equation
% Y[n] = C*X[n] + e
%-----------------------------
% n = Nº States
% m = Nº of inputs
% p = Nº of outputs
%
% See the IMPACT Deliverable 4 report for more detail on derivation of the
% Extended Kalman Filter
%
%%%%%%%%%%%%%%%%%%%%%%%%%%%%%%%%%%%%%%%%%%%%%%%%%%%%%%%%%%%%%%%%%%%%%%%%%

% Matrices of the system: A, B, C

persistent A B C P_k_k R1 R2 X_k_k bInit rFrequency rTimeStep rPhi0 rPhi0Star

% On the first step bInit is empty and so the initialisation can run

if isempty(bInit)
    
    bInit = 1;
    rFrequency = arEkfInitialisation(1);%0.5;
    rPhi0 = arEkfInitialisation(2);%1e5;
    rPhi0Star = arEkfInitialisation(3);%0;
    rTimeStep = arEkfInitialisation(4);
    
    A = zeros(3);
    A(1,:) = [cos(rFrequency*rTimeStep), sin(rFrequency*rTimeStep),...
        (-sin(rFrequency*rTimeStep)*rPhi0+cos(rFrequency*rTimeStep)*rPhi0Star)*rTimeStep];
    A(2,:) = [-sin(rFrequency*rTimeStep), cos(rFrequency*rTimeStep),...
        (-cos(rFrequency*rTimeStep)*rPhi0-sin(rFrequency*rTimeStep)*rPhi0Star)*rTimeStep];
    A(3,3) = 1;
    
    B = ones(3,1);
    C = zeros(1,3);
    C(1)=1;
      
    % Process noise covariance matrix
    R1 = [arEkfInitialisation(5),0,0;...
        0,arEkfInitialisation(6),0;...
        0,0,arEkfInitialisation(7)];
    
    % Measurement Noise covariance matrix
    R2 = arEkfInitialisation(8);
       
    P_k_k =  [arEkfInitialisation(9),0,0;...
        0,arEkfInitialisation(10),0;...
        0,0,arEkfInitialisation(11)];
    X_k_k = [rPhi0,rPhi0Star,rFrequency]';
    
    
end % End of initialisation

% No "input" for this EKF
U = 0;

% Time step consistent with simulation
rTimeStep = arEkfInitialisation(4);

% Define the A matrix as per deliverable 4 report
A(1,:) = [cos(rFrequency*rTimeStep) sin(rFrequency*rTimeStep) 0];
A(2,:) = [-sin(rFrequency*rTimeStep) cos(rFrequency*rTimeStep) 0];
A(3,3) = 1;


% Define the Jacobian as per deliverable 4 report - Note that for very
% small frequencies infinity must be avoided
JA = zeros(3);

if rFrequency<0.001 & rFrequency>=-0.001
    JA(1,:) = [cos(rFrequency*rTimeStep) sin(rFrequency*rTimeStep) rPhi0Star*rTimeStep-rPhi0*rFrequency*rTimeStep^2/2];
    JA(2,:) = [-sin(rFrequency*rTimeStep) cos(rFrequency*rTimeStep) -rPhi0*rTimeStep-rPhi0Star*rFrequency*rTimeStep^2/2];
    JA(3,3) = 1;
else
    JA(1,:) = [cos(rFrequency*rTimeStep) sin(rFrequency*rTimeStep) rPhi0Star*sin(rFrequency*rTimeStep)/rFrequency-rPhi0*(1-cos(rFrequency*rTimeStep))/rFrequency];
    JA(2,:) = [-sin(rFrequency*rTimeStep) cos(rFrequency*rTimeStep) -rPhi0*sin(rFrequency*rTimeStep)/rFrequency-rPhi0Star*(1-cos(rFrequency*rTimeStep))/rFrequency];
    JA(3,3) = 1;
end

% Define B and C Matrices
B = ones(3,1);
C = zeros(1,3);
C(1)=1;

% Kalman Filter
%---------------------------------
% Prediction
X_k1_k = A*X_k_k + B*U;

P_k1_k = JA*P_k_k*JA' + R1;

% Filter
Kf = P_k1_k*C'/(C*P_k1_k*C' + R2);
X_k1_k1 = X_k1_k + Kf*(rEstimatedExcitationForce-C*X_k1_k);
P_k1_k1 = P_k1_k - Kf*(C*P_k1_k*C'+R2)*Kf';


P_k_k = P_k1_k1; % for next cycle;
X_k_k = X_k1_k1; % for next cycle;

rFrequency = X_k_k(3);
rPhi0 = X_k_k(1);
rPhi0Star = X_k_k(2);

rFrequencyOutput = X_k_k(3);
rPhi0Output = X_k_k(1);
rPhi0StarOutput = X_k_k(2);

rAmplitudeOutput = sqrt(rPhi0.^2+rPhi0Star.^2);
